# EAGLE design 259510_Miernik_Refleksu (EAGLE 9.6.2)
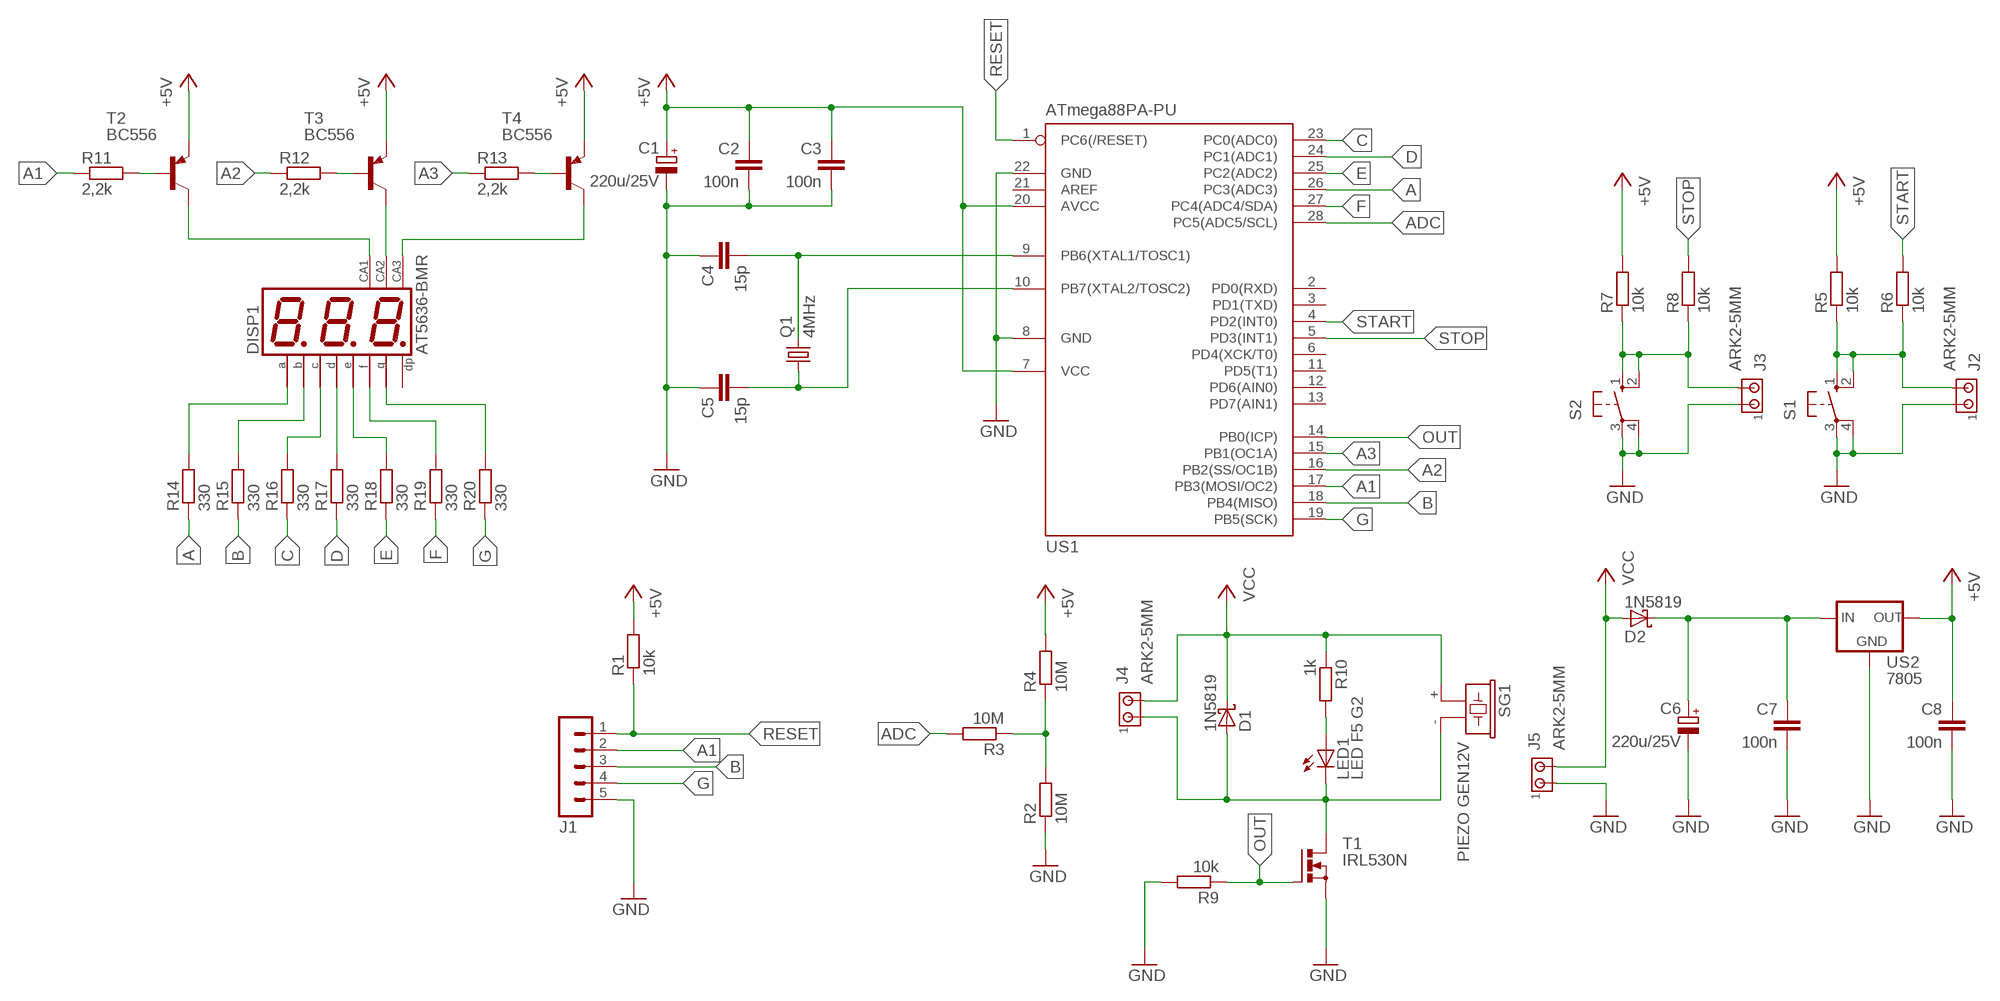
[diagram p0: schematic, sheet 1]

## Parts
C1  220u/25V  CPOL-EUE2.5-7  [E2,5-7]
C2  100n  C-EU050-025X075  [C050-025X075]
C3  100n  C-EU050-025X075  [C050-025X075]
C4  15p  C-EU050-025X075  [C050-025X075]
C5  15p  C-EU050-025X075  [C050-025X075]
C6  220u/25V  CPOL-EUE2.5-7  [E2,5-7]
C7  100n  C-EU050-025X075  [C050-025X075]
C8  100n  C-EU050-025X075  [C050-025X075]
D1  1N5819  1N5819-B  [DO41-7.6]
D2  1N5819  1N5819-B  [DO41-7.6]
DISP1  AT5636-BMR  BA56-12EWA  [BX56-12]
J1  MA05-1  [MA05-1]
J2  ARK2-5MM  [2PIN-5MM]
J3  ARK2-5MM  [2PIN-5MM]
J4  ARK2-5MM  [2PIN-5MM]
J5  ARK2-5MM  [2PIN-5MM]
LED1  LED F5 G2  LED5MM  [LED5MM]
Q1  4MHz  CRYSTALHC49U-V  [HC49U-V]
R1  10k  R-EU_0207/7  [0207/7]
R2  10M  R-EU_0207/7  [0207/7]
R3  10M  R-EU_0207/7  [0207/7]
R4  10M  R-EU_0207/7  [0207/7]
R5  10k  R-EU_0207/7  [0207/7]
R6  10k  R-EU_0207/7  [0207/7]
R7  10k  R-EU_0207/7  [0207/7]
R8  10k  R-EU_0207/7  [0207/7]
R9  10k  R-EU_0207/7  [0207/7]
R10  1k  R-EU_0207/7  [0207/7]
R11  2,2k  R-EU_0207/7  [0207/7]
R12  2,2k  R-EU_0207/7  [0207/7]
R13  2,2k  R-EU_0207/7  [0207/7]
R14  330  R-EU_0207/7  [0207/7]
R15  330  R-EU_0207/7  [0207/7]
R16  330  R-EU_0207/7  [0207/7]
R17  330  R-EU_0207/7  [0207/7]
R18  330  R-EU_0207/7  [0207/7]
R19  330  R-EU_0207/7  [0207/7]
R20  330  R-EU_0207/7  [0207/7]
S1  40-XX  [B3F-40XX]
S2  40-XX  [B3F-40XX]
SG1  PIEZO GEN12V  F/CM12P  [F/CM12P]
T1  IRL530N  BUZ11BH  [TO220BH]
T2  BC556  [TO92-EBC]
T3  BC556  [TO92-EBC]
T4  BC556  [TO92-EBC]
US1  ATmega88PA-PU  MEGA8-P  [DIL28-3]
US2  7805  78XXL  [78XXL]

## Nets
+5V: C1.+ C2.1 C3.1 C8.1 R1.2 R4.2 R5.2 R7.2 T2.E T3.E T4.E US1.7(VCC) US1.20(AVCC) US2.OUT
A: R14.1 US1.26(PC3(ADC3))
A1: J1.2 R11.1 US1.17(PB3(MOSI/OC2))
A2: R12.1 US1.16(PB2(SS/OC1B))
A3: R13.1 US1.15(PB1(OC1A))
ADC: R3.2 US1.28(PC5(ADC5/SCL))
B: J1.3 R15.1 US1.18(PB4(MISO))
C: R16.1 US1.23(PC0(ADC0))
D: R17.1 US1.24(PC1(ADC1))
E: R18.1 US1.25(PC2(ADC2))
F: R19.1 US1.27(PC4(ADC4/SDA))
G: J1.4 R20.1 US1.19(PB5(SCK))
GND: C1.- C2.2 C3.2 C4.1 C5.1 C6.- C7.2 C8.2 J1.5 J2.P$1 J3.P$1 J5.P$1 R2.1 R9.2 S1.3(P) S1.4(P1) S2.3(P) S2.4(P1) T1.S US1.8(GND) US1.22(GND) US2.GND
N$1: R2.2 R3.1 R4.1
N$2: C6.+ C7.1 D2.C US2.IN
N$3: C5.2 Q1.1 US1.10(PB7(XTAL2/TOSC2))
N$4: C4.2 Q1.2 US1.9(PB6(XTAL1/TOSC1))
N$6: J2.P$2 R5.1 R6.1 S1.1(S) S1.2(S1)
N$7: J3.P$2 R7.1 R8.1 S2.1(S) S2.2(S1)
N$8: LED1.A R10.2
N$11: R11.2 T2.B
N$12: R12.2 T3.B
N$13: R13.2 T4.B
N$14: DISP1.9(CA) T3.C
N$17: D1.A J4.P$1 LED1.K(C) SG1.- T1.D
N$18: DISP1.12(CA) T2.C
N$19: DISP1.8(CA) T4.C
N$21: DISP1.2(D) R17.2
N$22: DISP1.4(C) R16.2
N$23: DISP1.1(E) R18.2
N$24: DISP1.10(F) R19.2
N$25: DISP1.5(G) R20.2
N$26: DISP1.7(B) R15.2
N$27: DISP1.11(A) R14.2
OUT: R9.1 T1.G US1.14(PB0(ICP))
RESET: J1.1 R1.1 US1.1(PC6(/RESET))
START: R6.2 US1.4(PD2(INT0))
STOP: R8.2 US1.5(PD3(INT1))
VCC: D1.C D2.A J4.P$2 J5.P$2 R10.1 SG1.+
Unconnected: DISP1.3(DP) US1.2(PD0(RXD)) US1.3(PD1(TXD)) US1.6(PD4(XCK/T0)) US1.11(PD5(T1)) US1.12(PD6(AIN0)) US1.13(PD7(AIN1)) US1.21(AREF)

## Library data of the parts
C1 C6 = rcl:CPOL-EU: POLARIZED CAPACITOR, European symbol
C2-C5 C7 C8 = rcl:C-EU: CAPACITOR, European symbol
D1 D2 = diode:1N581*: 1.0A SCHOTTKY BARRIER RECTIFIER
DISP1 = display-kingbright:B?56-12*WA: 14.22mm (0.56INCH) THREE DIGIT NUMERIC DISPLAY Source: http://www.kingbright.com .. BA56-11EWA(Ver1189474895.pdf
J1 = zlacza_futrzak:MA05-1: PIN HEADER; OC_FARNELL: unknown; OC_NEWARK: unknown
J2-J5 = zlacza_futrzak:ARK2: ARK 2
LED1 = led:LED: LED
Q1 = crystal:CRYSTAL: CRYSTAL; OC_FARNELL: 1666969; OC_NEWARK: unknown
R1-R20 = rcl:R-EU_: RESISTOR, European symbol
S1 S2 = switch-omron:40-XX: OMRON SWITCH; MF: OMRON COMPONENTS USA; MPN: B3F-4000; OC_FARNELL: 176434; OC_NEWARK: 36K3105
SG1 = buzzer:F/CM12P: BUZZER; OC_FARNELL: unknown; OC_NEWARK: unknown
T1 = transistor-power:BUZ11: N-CHANNEL MOS FET
T2-T4 = transistor-pnp:BC556*: PNP Transistror
US1 = atmel:MEGA8-P: MICROCONTROLLER 8 Kbytes FLASH, 1 kbytes SRAM, 512 bytes EEPROM, USART, 4-channel 10 bit ADC, 2-channel 8 bit ADC Pin compatible with Atmega48, ATMega88, ATMega168 Source: avr.lbr; OC_FARNELL: unknown; OC_NEWARK: unknown
US2 = v-reg:78XXL: VOLTAGE REGULATOR

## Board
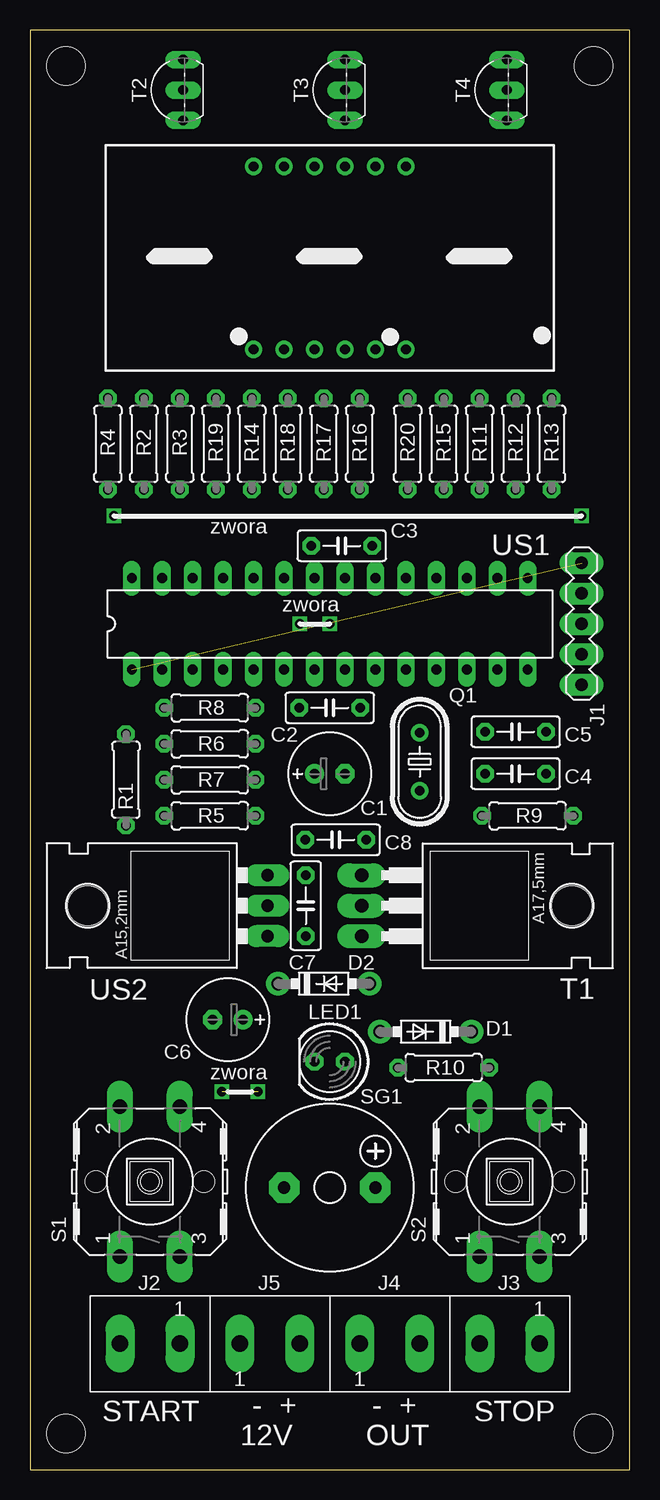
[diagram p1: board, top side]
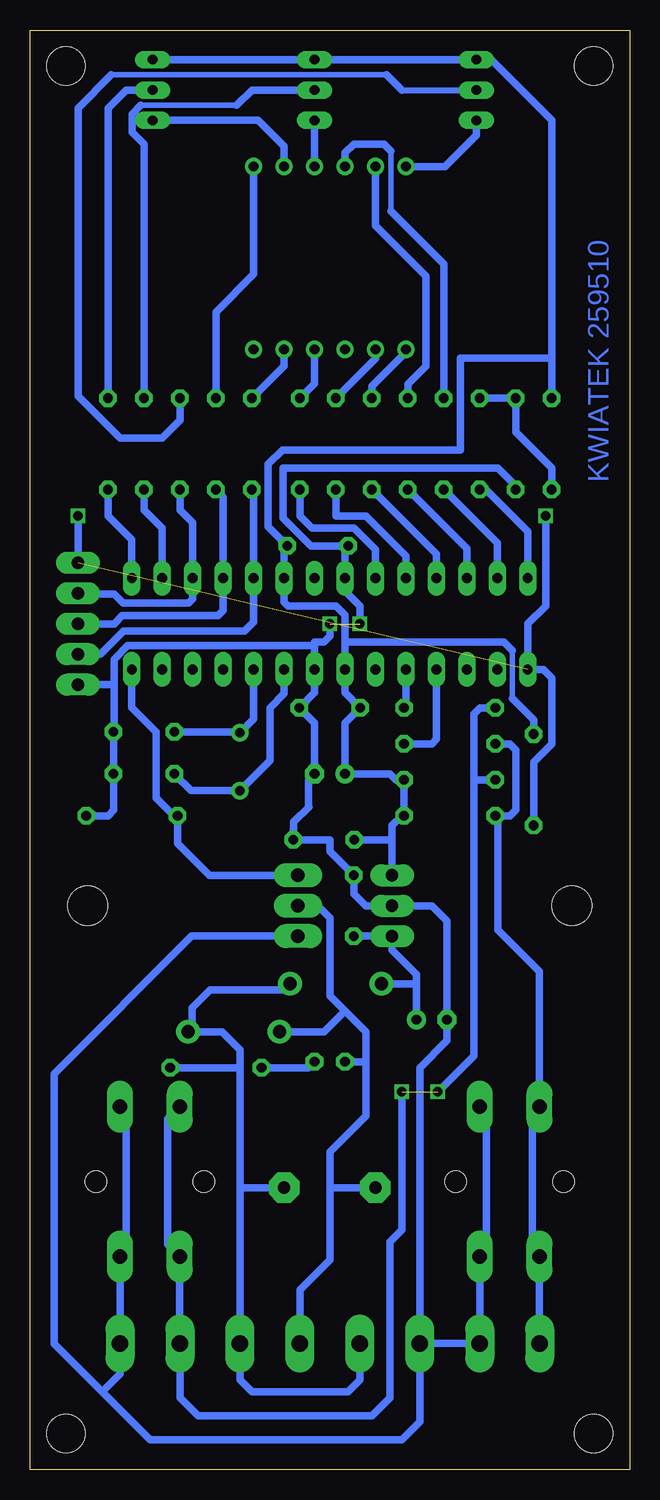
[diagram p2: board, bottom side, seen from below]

Size 50 x 120 mm. Coordinates in mm from the lower left corner, seen from the top.
Outline: 0,0 50,0 50,120 0,120 0,0
Copper layers (1*16): Top 0.035mm / dielectric 1.5mm / Bottom 0.035mm
Design rules "default *": minimum track width 24mil, minimum drill 0.8mm, track to track 12mil, track to pad 12mil, pad to pad 8mil, via to via 8mil, smd to smd 8mil, copper to edge 40mil, drill to drill 8mil, minimum pad ring 10mil, minimum via ring 8mil, stop-mask expansion 4mil, vias tented up to drill 0mil, thermal gap 10mil
Holes 3.2 mm at 3,117 47,117 3,3 47,3

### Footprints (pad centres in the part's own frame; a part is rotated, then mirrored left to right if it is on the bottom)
E2,5-7 = drill 0.813 pad 1.6: + -1.27,0 | drill 0.813 pad 1.6 octagon: - 1.27,0
C050-025X075 = drill 0.813 octagon: 1 -2.54,0; 2 2.54,0
DO41-7.6 = drill 1.1 pad 1.7: A 3.81,0; C -3.81,0
BX56-12 = drill 0.8 pad 1.422: 1 -6.35,-7.62; 2 -3.81,-7.62; 3 -1.27,-7.62; 4 1.27,-7.62; 5 3.81,-7.62; 6 6.35,-7.62; 7 6.35,7.62; 8 3.81,7.62; 9 1.27,7.62; 10 -1.27,7.62; 11 -3.81,7.62; 12 -6.35,7.62
MA05-1 = drill 1.016 long: 1 -5.08,0; 2 -2.54,0; 3 0,0; 4 2.54,0; 5 5.08,0
2PIN-5MM = drill 1.4 long: P$1 -2.5,0; P$2 2.5,0
LED5MM = drill 0.813 octagon: A -1.27,0; K 1.27,0
HC49U-V = drill 0.813: 1 -2.413,0; 2 2.413,0
0207/7 = drill 0.813 octagon: 1 -3.81,0; 2 3.81,0
B3F-40XX = drill 1.194 long: 1 -6.248,2.489; 2 6.248,2.489; 3 -6.248,-2.489; 4 6.248,-2.489 | hole 1.803: 0,-4.496; 0,4.496
F/CM12P = drill 1.016 pad 2.54 octagon: + 3.81,0; - -3.81,0
TO220BH = drill 1.118 long: D 0,-6.35; G -2.54,-6.35; S 2.54,-6.35 | hole 3.302: 0,11.176
TO92-EBC = drill 0.813 long: B 0,-1.27; C -2.54,-1.27; E 2.54,-1.27
DIL28-3 = drill 0.813 long: 1 -16.51,-3.81; 2 -13.97,-3.81; 3 -11.43,-3.81; 4 -8.89,-3.81; 5 -6.35,-3.81; 6 -3.81,-3.81; 7 -1.27,-3.81; 8 1.27,-3.81; 9 3.81,-3.81; 10 6.35,-3.81; 11 8.89,-3.81; 12 11.43,-3.81; 13 13.97,-3.81; 14 16.51,-3.81; 15 16.51,3.81; 16 13.97,3.81; 17 11.43,3.81; 18 8.89,3.81; 19 6.35,3.81; 20 3.81,3.81; 21 1.27,3.81; 22 -1.27,3.81; 23 -3.81,3.81; 24 -6.35,3.81; 25 -8.89,3.81; 26 -11.43,3.81; 27 -13.97,3.81; 28 -16.51,3.81
78XXL = drill 1.016 long: GND 0,-3.81; IN -2.54,-3.81; OUT 2.54,-3.81 | hole 3.302: 0,11.176

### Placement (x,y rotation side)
C1  25,58 0 top
C2  25,63.5 0 top
C3  26,77 180 top
C4  40.5,58 180 top
C5  40.5,61.5 180 top
C6  16.5,37.5 180 top
C7  23,47 90 top
C8  25.5,52.5 0 top
D1  33,36.5 180 top
D2  24.5,40.5 0 top
DISP1  25,101 0 top
J1  46,70.5 270 top
J2  10,10.5 180 top
J3  40,10.5 180 top
J4  30,10.5 0 top
J5  20,10.5 0 top
LED1  25,34 180 top
Q1  32.5,59 270 top
R1  8,57.5 90 top
R2  9.5,85.5 90 top
R3  12.5,85.5 270 top
R4  6.5,85.5 90 top
R5  15,54.5 0 top
R6  15,60.5 0 top
R7  15,57.5 0 top
R8  15,63.5 0 top
R9  41.5,54.5 0 top
R10  34.5,33.5 180 top
R11  37.5,85.5 90 top
R12  40.5,85.5 90 top
R13  43.5,85.5 90 top
R14  18.5,85.5 90 top
R15  34.5,85.5 90 top
R16  27.5,85.5 90 top
R17  24.5,85.5 90 top
R18  21.5,85.5 90 top
R19  15.5,85.5 90 top
R20  31.5,85.5 90 top
S1  10,24 90 top
S2  40,24 90 top
SG1  25,23.5 0 top
T1  34,47 270 top
T2  11.5,115 90 top
T3  25,115 90 top
T4  38.5,115 90 top
US1  25,70.5 0 top
US2  16,47 90 top

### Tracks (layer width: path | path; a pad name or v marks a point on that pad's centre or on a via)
+5V
  Bottom 0.44: 9.76,64.26 9.76,68.26
  Bottom 0.61: T4.E T3.E T2.E 11.54,117.54 6.5,112.5 6.5,92.66 | 6.5,92.66 R4.2 | 6.5,92.66 14.09,92.66 14.09,85 28.94,85 30.14,83.81 30.14,78.6 C3.1 28.81,76.73 US1.20 28.81,72.31 28.5,72 24.5,72 23.73,71.23 23.73,69 | 23.73,69 US1.7 23.73,64.77 C2.1 23.73,62.23 C1.+ 20,58 19.5,57.5 R7.2 R5.2 19,54.5 19.81,53.69 19.81,52.5 | R1.2 8,62.5 9.76,64.26 | 9.76,68.26 10.5,69 23.73,69 | US2.OUT 19.81,52.5 | C8.1 19.81,52.5
A
  Bottom 0.61: US1.26 13.57,76.76 R14.1
A1
  Bottom 0.61: R11.1 37.5,80 36.43,78.93 US1.17 36.43,72.57 36.77,72.23 42.23,72.23 43,73 45.96,73 J1.2
A2
  Bottom 0.61: US1.16 38.97,78.47 40.5,80 R12.1
A3
  Bottom 0.61: US1.15 41.51,77.51 43.5,79.5 R13.1
ADC
  Bottom 0.61: US1.28 8.49,78.18 12,81.69 R3.2
B
  Bottom 0.61: R15.1 33.89,81.08 US1.18 33.89,71.61 34.3,71.2 42.3,71.2 43,70.5 J1.3
C
  Bottom 0.61: US1.23 21.19,76.69 23,78.5 26.5,78.5 27.5,79.5 R16.1
D
  Bottom 0.61: US1.24 18.65,76.15 22,79.5 24.5,79.5 R17.1
E
  Bottom 0.61: US1.25 16.11,76.3 R18.1
F
  Bottom 0.61: US1.27 11.03,77.22 R19.1
G
  Bottom 0.61: R20.1 31.35,81.54 US1.19 31.35,70.65 32.1,69.9 42.2,69.9 44.1,68 45.96,68 J1.4
GND  (via drill 0.8)  (1 unrouted)
  Bottom 0.61: R2.1 9.5,82 11,83.5 28.91,83.5 28.91,79.33 26.58,77 C3.2 23.73,76.73 US1.22 23.73,73.23 22.5,72 v22.5,70.5 | J1.5 43.08,65.42 43,65.5 | 26.27,68.67 41.85,68.67 43,67.52 43,65.5 | 26.27,68.67 US1.8 26.27,64.77 C2.2 26.27,62.23 C1.- 26.77,57.5 26.77,55.27 26.75,55.25 28.04,53.96 C8.2 25,52.5 25,51.54 C7.2 23,48 22,47 US2.GND 16.5,47 15.23,45.73 C6.- 15.23,35.77 17.5,33.5 J5.P$1 | 26.27,68.67 26.27,69 25.5,69 25,69.5 v25,70.5 | R9.2 43.5,54.5 43.04,54.96 C4.1 C5.1 43,61.54 43,65.5 | T1.S 36.54,44.46 48,33 48,10.5 44,6.5 | J5.P$1 17.5,4 19,2.5 40,2.5 44,6.5 | J2.P$1 J5.P$1 | J2.P$1 S1.3 11.93,18.31 11.93,29.69 S1.4 | J2.P$1 | S2.4 41.99,29.75 41.99,18.25 S2.3 J3.P$1 42.5,8 44,6.5
N$1
  Bottom 0.61: R3.1 R2.2 9.5,86.5 6.5,83.5 R4.1
N$2
  Bottom 0.61: C7.1 US2.IN 19.81,43.31 17.77,41.27 17.77,40.5 | C6.+ 17.77,40.5 | D2.C 17.77,40.5
N$3
  Bottom 0.61: C5.2 32.59,61.5 Q1.1 31.35,62.56 US1.10
N$4
  Bottom 0.61: US1.9 28.81,64.69 30,63.5 30,59.09 Q1.2 36.55,56.59 C4.2
N$6
  Bottom 0.61: R6.1 10,60.5 9.5,60 9.5,55 10,54.5 R5.1 11,54.31 11,45 7.51,41.51 S1.2 8.12,29.64 8.12,18.36 S1.1 J2.P$2
N$7  (via drill 0.8)  (1 unrouted)
  Bottom 0.61: R8.1 12.5,63.5 13,63 13,57.5 | 13,57.5 R7.1 | 13,57.5 13,34.5 v16,31.5 | S2.1 | S2.2 38.51,29.25 38.51,18.75 S2.1 | S2.1 37.51,10.51 J3.P$2 37.5,6 36,4.5 21.5,4.5 20,6 20,19 19,20 v19,31.5
N$8
  Bottom 0.61: R10.2 26.77,33.5 LED1.A
N$11
  Bottom 0.44: 43.22,116.28 20.28,116.28
  Bottom 0.508: 19,115 T2.B
  Bottom 0.61: R11.2 37.5,87.5 39,86 42.5,86 46,89.5 46,113.5 43.22,116.28 | 20.28,116.28 19,115
N$12
  Bottom 0.44: 40.77,113.73 32.77,113.73
  Bottom 0.61: R12.2 40.5,110.5 41.5,111.5 41.5,113 40.77,113.73 | 32.77,113.73 31.5,115 T3.B
N$13
  Bottom 0.61: R13.2 43.5,113.5 42,115 T4.B
N$14
  Bottom 0.61: DISP1.9 T3.C
N$17
  Bottom 0.61: T1.D 26,47 25,46 25,41 25,39.5 23.75,38.25 | 23.75,38.25 22,36.5 22,34 | 22,34 22,29.5 25,26.5 25,23.5 | 25,23.5 25,17.5 27.5,15 J4.P$1 | D1.A 25.5,36.5 23.75,38.25 | LED1.K 22,34 | SG1.- 25,23.5
N$18
  Bottom 0.61: T2.C 12.77,111.23 15.38,108.62 DISP1.12
N$19
  Bottom 0.61: DISP1.8 28.81,110.31 30.96,112.46 T4.C
N$21
  Bottom 0.61: R17.2 21.19,92.62 DISP1.2
N$22
  Bottom 0.61: R16.2 26.27,90.54 DISP1.4
N$23
  Bottom 0.61: R18.2 21.5,90.31 18.65,93.16 DISP1.1
N$24
  Bottom 0.44: 19.91,104.91 19.91,109.91
  Bottom 0.61: R19.2 15.5,100.5 19.91,104.91 | 19.91,109.91 20.5,110.5 23,110.5 23.73,109.77 DISP1.10
N$25
  Bottom 0.61: R20.2 28.81,92 DISP1.5
N$26
  Bottom 0.61: R15.2 34.5,96.5 31.35,99.65 DISP1.7
N$27
  Bottom 0.61: R14.2 18.5,90.5 17,92 17,99.5 21.19,103.69 DISP1.11
OUT
  Bottom 0.61: US1.14 41.51,63.51 39.5,61.5 39.5,56 38,54.5 R9.1 37.69,52.19 35.04,49.54 T1.G
RESET  (via drill 0.8)  (1 unrouted)
  Bottom 0.61: v7,79.5 7,72 8.49,70.51 US1.1 7.19,66.69 6.5,66 6.5,60.5 8,59 R1.1 | v46,79.5 J1.1
START
  Bottom 0.61: US1.4 16.11,60.89 16.5,60.5 R6.2
STOP
  Bottom 0.61: US1.5 18.65,63.66 R8.2
VCC
  Bottom 0.61: J5.P$2 22.5,7.5 23.5,6.5 31.5,6.5 32.5,7.5 J4.P$2 32.5,23.5 | 32.5,23.5 32.5,33.5 | 32.5,33.5 32.5,35 34,36.5 36.5,36.5 | 36.5,36.5 D1.C | SG1.+ 32.5,23.5 | R10.1 32.5,33.5 | D2.A 28.81,40 35,40 36.5,38.5 36.5,36.5

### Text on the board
Bottom: KWIATEK 259510
tPlace: zwora | zwora | zwora | START | - + | - + | STOP | 12V | OUT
